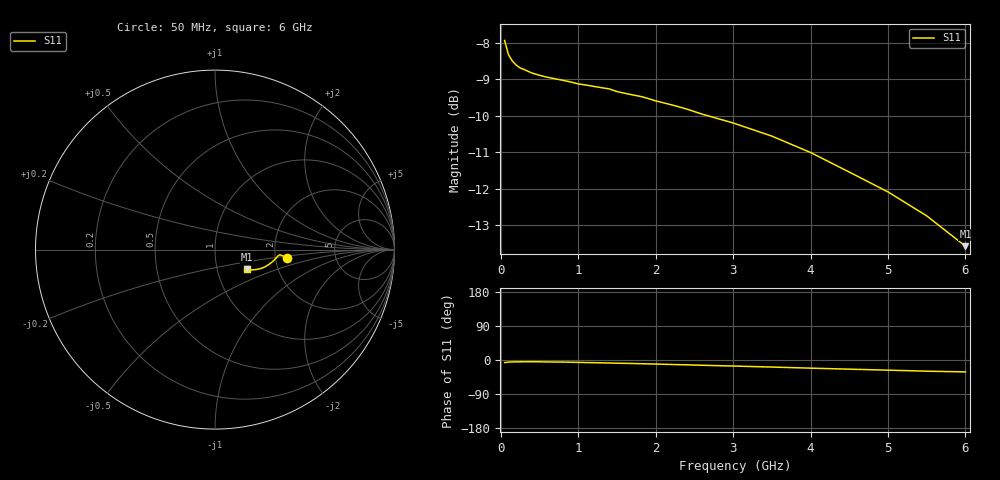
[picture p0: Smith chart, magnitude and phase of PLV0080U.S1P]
! Infineon Technologies  Discrete & RF Semiconductors
! BAR 64-04W /-05W /-06W
! Si PIN Diode in SOT323
! IF = 0.08 mA
! S-Parameters:  October  2008
# GHz  S  MA  R  50
!  f  S11
! GHz  MAG  ANG
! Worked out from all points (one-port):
!   34 points, 50 MHz to 6 GHz, reference 50 ohm
!   lowest |S11| = -13.6 dB at 6 GHz (marker M1), VSWR 1.53, Z = 69.6 - j15.9 ohm
!   |S11| at or under -10 dB: 2.677 GHz to end of sweep
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0.05  0.4014 -6.7
0.1  0.3836 -5.6
0.15  0.3761 -5.1
0.2  0.3713 -4.9
0.25  0.368 -4.8
0.3  0.3662 -4.7
0.4  0.3622 -4.6
0.5  0.3595 -4.8
0.6  0.3574 -5.1
0.8  0.3539 -5.5
1  0.3499 -6.3
1.4  0.3444 -7.9
1.5  0.3415 -8.4
1.6  0.3397 -8.8
1.7  0.3379 -9.2
1.8  0.3364 -9.7
1.9  0.3342 -10.3
2  0.3316 -10.7
2.2  0.3276 -11.8
2.4  0.3231 -12.8
2.6  0.3179 -13.9
3  0.3092 -15.9
3.5  0.2966 -18.6
4  0.2816 -21.5
4.5  0.2647 -24.2
5  0.2486 -26.8
5.5  0.2304 -29.5
6  0.2094 -31.4
